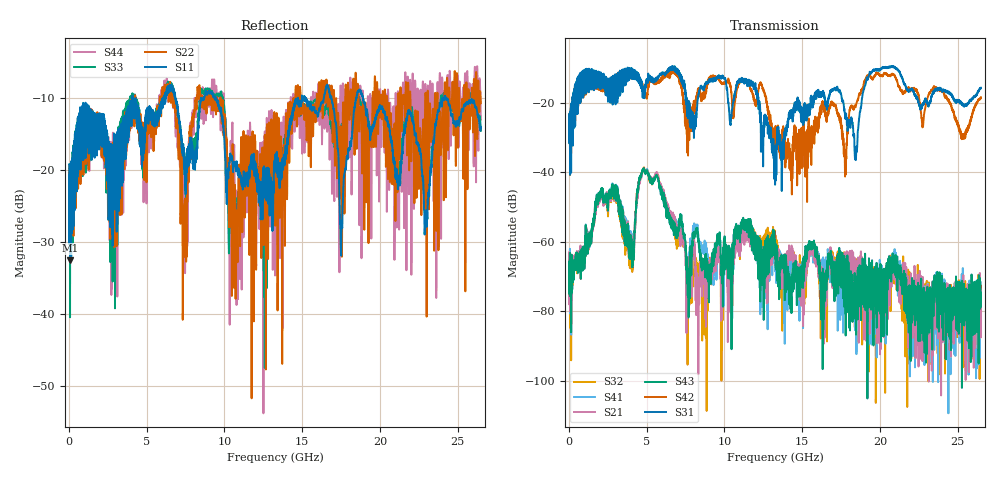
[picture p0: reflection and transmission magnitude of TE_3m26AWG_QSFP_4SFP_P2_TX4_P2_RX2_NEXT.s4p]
!Agilent Technologies,N5222A,MY51421691,A.10.00.00
!Agilent N5222A: A.10.00.00
!Date: Friday, January 30, 2015 12:35:40
!Correction: S11(Full 4 Port(1,2,3,4))
!S12(Full 4 Port(1,2,3,4))
!S13(Full 4 Port(1,2,3,4))
!S14(Full 4 Port(1,2,3,4))
!S21(Full 4 Port(1,2,3,4))
!S22(Full 4 Port(1,2,3,4))
!S23(Full 4 Port(1,2,3,4))
!S24(Full 4 Port(1,2,3,4))
!S31(Full 4 Port(1,2,3,4))
!S32(Full 4 Port(1,2,3,4))
!S33(Full 4 Port(1,2,3,4))
!S34(Full 4 Port(1,2,3,4))
!S41(Full 4 Port(1,2,3,4))
!S42(Full 4 Port(1,2,3,4))
!S43(Full 4 Port(1,2,3,4))
!S44(Full 4 Port(1,2,3,4))
!S4P File: Measurements: <S11,S12,S13,S14>,
!<S21,S22,S23,S24>,
!<S31,S32,S33,S34>,
!<S41,S42,S43,S44>:
# Hz S  dB  R 50.0
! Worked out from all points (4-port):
!   2650 points, 10 MHz to 26.5 GHz, reference 50 ohm
!   strongest paths, dB at 10 MHz, 6.63 GHz, 13.26 GHz, 19.88 GHz, 26.5 GHz:
!     S31: -25.0, -10.5, -43.6, -10.4, -15.7
!     S42: -24.8, -11.5, -30.6, -11.8, -18.5
!     S43: -70.1, -55.7, -64.9, -75.4, -74.9
!     S21: -63.1, -53.5, -63.2, -69.1, -77.1
!     S41: -73.3, -54.2, -68.5, -70.0, -78.3
!     S32: -71.1, -54.7, -59.1, -78.5, -72.7
!   lowest |S11| = -32.5 dB at 70 MHz (marker M1), VSWR 1.05, Z = 52.4 + j0.243 ohm
!   |S11| at or under -10 dB: start of sweep to 4.075 GHz; 9.454 GHz to 14.73 GHz (5.275 GHz wide, 43.6 % of centre); 18.91 GHz to 24.06 GHz (5.147 GHz wide, 24 % of centre)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
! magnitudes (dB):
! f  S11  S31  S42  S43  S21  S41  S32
! 10 MHz  -19.2  -25.0  -24.8  -70.1  -63.1  -73.3  -71.1
! 70 MHz  -32.5  -40.8  -40.8  -75.7  -73.7  -76.0  -73.0
! 4.05 GHz  -11.2  -11.4  -12.2  -63.4  -62.1  -60.6  -65.2
! 4.9 GHz  -12.7  -15.7  -18.1  -40.3  -39.9  -40.0  -40.2
! 8.81 GHz  -9.0  -14.5  -16.2  -65.3  -84.5  -63.3  -87.6
! 13.22 GHz  -18.7  -42.0  -29.3  -60.7  -61.4  -65.6  -59.6
! 26.5 GHz  -14.1  -15.7  -18.5  -74.9  -77.1  -78.3  -72.7
